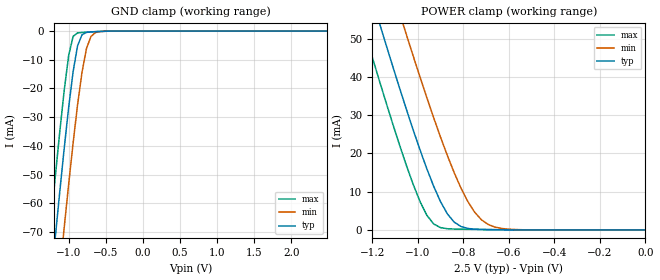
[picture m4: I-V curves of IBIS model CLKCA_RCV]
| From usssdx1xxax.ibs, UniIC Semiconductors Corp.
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|   Model CLKCA_RCV
[Model]  CLKCA_RCV
Model_type Input
Polarity   Non-Inverting
Vinl =   940.000mV
Vinh =   1.560V
C_comp   0.9200pF   0.8940pF   0.9290pF
[Temperature Range]   25.0000   0.1250k   -55.0000
[Voltage Range]   2.5000V   2.3000V   2.7000V
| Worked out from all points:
|   GND clamp passes 1 mA (typ) near -0.80 V on its own axis
|   POWER clamp passes 1 mA (typ) near -0.81 V on its own axis
[GND_clamp]
|Voltage   I(typ)   I(min)   I(max)
-2.5V     -448.9mA   -475.2mA   -429.8mA
-1.3V     -104.3mA   -132.5mA   -83.19mA
-1.24V    -87.9mA    -116.1mA   -66.74mA
-1.18V    -71.75mA   -99.93mA   -50.65mA
-1.06V    -40.81mA   -68.4mA    -20.62mA
-1V       -26.57mA   -53.3mA    -8.454mA
-940mV    -14.08mA   -38.91mA   -1.827mA
-880mV    -5.084mA   -25.64mA   -632.2uA
-820mV    -1.257mA   -14.27mA   -468.9uA
-760mV    -458.7uA   -6.041mA   -371.8uA
-640mV    -199.4uA   -526.4uA   -199.6uA
2.48V     17.21nA    15.6nA     2.243nA
[POWER_clamp]
|Voltage   I(typ)   I(min)   I(max)
-2.49V    329.6mA    347.9mA    316mA
-1.26V    72.27mA    92.03mA    57.21mA
-1.23V    66.27mA    86.05mA    51.18mA
-1.17V    54.42mA    74.19mA    39.31mA
-1.08V    37.13mA    56.76mA    22.24mA
-1.05V    31.57mA    51.07mA    16.91mA
-990mV    20.94mA    39.96mA    7.446mA
-930mV    11.43mA    29.33mA    1.577mA
-840mV    2.06mA     14.99mA    240.1uA
-720mV    124uA      2.655mA    125uA
-600mV    29.88uA    200.7uA    50.08uA
0V        18.39nA    1.604nA    4.78nA
